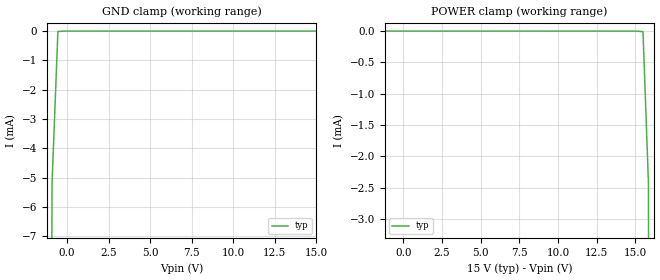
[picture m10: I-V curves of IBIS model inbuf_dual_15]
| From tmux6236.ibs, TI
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| inbuf_dual_15
[Model]   inbuf_dual_15
Model_type   Input
Vinl = 0.8
Vinh = 1.3
|   typ   min   max
C_comp   4.014581e-13   NA   NA
[Voltage Range]   15   NA   NA
[Temperature Range]   27   NA   NA
[Power Clamp Reference]   15   NA   NA
[GND Clamp Reference]   0   NA   NA
[GND Clamp]
|   Voltage   I(typ)   I(min)   I(max)
-20V      -5.936A    NA         NA
-1.263V   -72.13mA   NA         NA
-909.1mV  -5.222mA   NA         NA
-555.6mV  -13.12uA   NA         NA
15V       971.3nA    NA         NA
[POWER Clamp]
|   Voltage   I(typ)   I(min)   I(max)
-5V       1.194uA    NA         NA
15.51V    -7.828uA   NA         NA
15.86V    -2.444mA   NA         NA
16.21V    -58.83mA   NA         NA
30V       -4.366A    NA         NA
